TYPE ST_Parameter_HomeConfig :
STRUCT
	HomeMode 			: E_HomeMode   	:= E_HomeMode.ABSOLUTESWITCH;(* 寻参模式*)
	EnableZpulseHome	: BOOL;			(* 补充Z脉冲回零*)
	
	PositiveSwitch 		: BOOL;			(* 正限位信号*)
	NegativeSwitch		: BOOL;			(* 负限位信号*)
	RefrenceSignal		: BOOL;			(* 原点信号*)
	HomeVelocity		: LREAL := 3;	(* 回零速度*)
	HomeVelocityCorrect	: LREAL := 0.1;	(* 回零矫正速度 - 从homeoffset返回0位置速度*)
	HomeZPulseVelocity	: LREAL := 0.1;	(* 寻Z脉冲速度*)
	HomeOffset			: LREAL;		(* 回零偏置*)
	Acceleration		: LREAL;		(* 加速度*)
	Deceleration		: LREAL;		(* 减速度*)
	Jerk				: LREAL;		(* 加加速*)

	BlockHomeDetectionVeloLimit	: LREAL := 1;		(* 堵转回零 - 判断停转的速度限制 *)
	BlockHomeDetectionVeloTime	: TIME  := T#500MS; (* 堵转回零 - 判断停转的速度限制时间 *)
	BlockHomeTimeLimit			: TIME	:= T#100S;	(* 堵转回零 - 回零时间限制 *)
	BlockHomeDistanceLimit		: LREAL := 3000;	(* 堵转回零 - 回零距离限制 *)
	BlockHomeTorqueLimit		: LREAL := 20;		(* 堵转回零 - 回零扭矩限制 单位额定扭矩百分比 *)
	BlockHomeLagLimit			: LREAL := 5;		(* 堵转回零 - 回零堵转后跟随误差限制 *)
	
	(* 回零开始方向 *)
	StartDirection	: MC_Home_Direction		:= MC_Home_Direction.mcSwitchPositive;
	(* 寻Z脉冲的方向，选择mcNegativeDirection反方向 mcPositiveDirection为正方向*)
	ZPulseDirection	: MC_Home_Direction		:= MC_Home_Direction.mcPositiveDirection;;
	(* 目标信号的边缘 *)
	SwitchMode		: MC_Switch_Mode		:= MC_Switch_Mode.mcEdgeSwitchPositive; 

END_STRUCT
END_TYPE
